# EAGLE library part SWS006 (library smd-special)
SMD Dip Switch 6 pol.
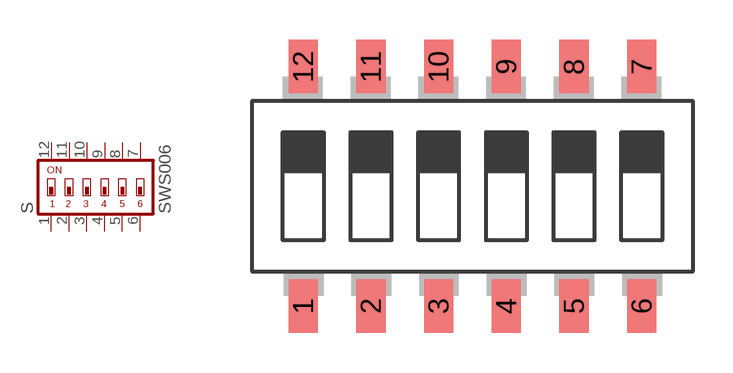
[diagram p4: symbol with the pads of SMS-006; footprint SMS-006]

Designator prefix S

## SWS006  [SMS-006]
1  1  pas
2  2  pas
3  3  pas
4  4  pas
5  5  pas
6  6  pas
7  7  pas
8  8  pas
9  9  pas
10  10  pas
11  11  pas
12  12  pas

## Footprint SMS-006 (pad centres in mm)
DIP SWITCH
smd 1.092 x 2.007: 1 -6.35,-4.496; 2 -3.81,-4.496; 3 -1.27,-4.496; 4 1.27,-4.496; 5 3.81,-4.496; 6 6.35,-4.496; 7 6.35,4.496; 8 3.81,4.496; 9 1.27,4.496; 10 -1.27,4.496; 11 -3.81,4.496; 12 -6.35,4.496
